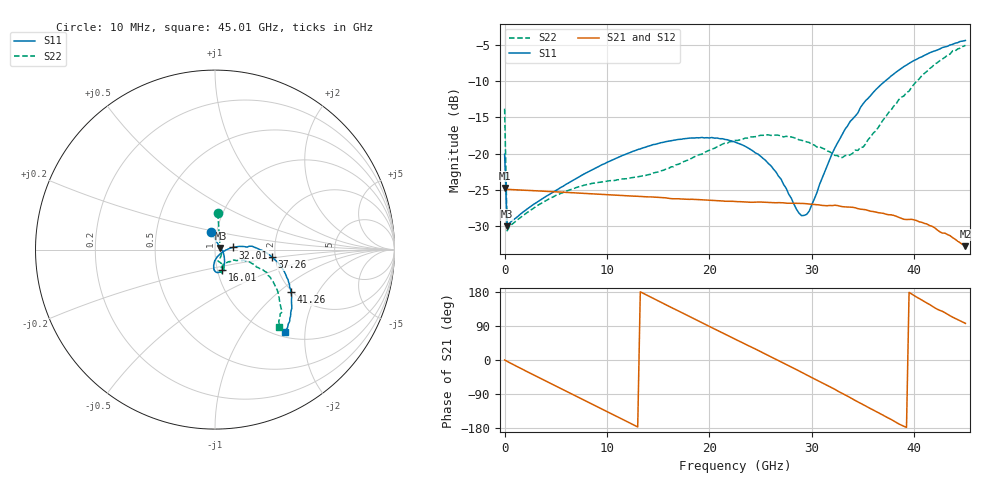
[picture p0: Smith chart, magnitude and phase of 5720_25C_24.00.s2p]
! Device:  ADRF5720
! Description: 0.5dB LSB GaAs MMIC 6-bit Digital Attenuator
! Frequency:  0.000009 -  40 GHz
! Ports:
!	RF1	= Port 1
!	RF2	= Port 2
! Vdd:  3.3 Volt
! Vss:  -3.3 Volt
! Control:  0/3.3 Volt
! State:  24.00 dB attenuation
! Data:  The device was measured using G-S-G Probes on a matrix board.
!  Data was collected using an calibrated 4 port network analyzer.
!  The reference plane for this measurement is at the launchers.
! Note:  Analog Devices supplies this data as a sample of measured data
!  for this product.  Your particular data for this product may vary.
!  Data was taken at 25 degrees C.
!  Analog Devices reserves the right to change this data at anytime.
# GHZ S DB R 45.0
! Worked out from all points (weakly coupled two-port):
!   181 points, 10 MHz to 45.01 GHz, reference 45 ohm
!   highest |S21| = -24.71 dB at 10 MHz (marker M1); lowest = -32.7 dB at 45.01 GHz (marker M2)
!   lowest |S11| = -30.0 dB at 260 MHz (marker M3), VSWR 1.07, Z = 47.8 + j0.88 ohm
!   |S11| at or under -10 dB: start of sweep to 37.17 GHz
!   |S22| runs from -30.6 to -5.1 dB; largest |S21 - S12| = 0.00012
!   S11 on the Smith chart (normalised r, x): 10 MHz: 0.94, +0.18; 16.01 GHz: 1.05, -0.25; 32.01 GHz: 1.22, +0.03; 37.26 GHz: 1.92, -0.18; 41.26 GHz: 1.97, -1.22; 45.01 GHz: 1.09, -1.57
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0.01  -20.08 103.8  -24.71 0.1  -24.71 0.1  -13.80 85.6
0.26  -30.01 16.9  -24.91 -3.8  -24.92 -3.8  -30.62 15.5
3.26  -26.59 -16.1  -25.12 -45.0  -25.13 -45.0  -27.10 -35.2
7.76  -22.80 -43.2  -25.47 -105.8  -25.47 -105.8  -24.35 -68.4
15.26  -18.49 -69.2  -26.04 152.5  -26.04 152.5  -22.38 -68.9
16.01  -18.28 -71.4  -26.14 142.2  -26.14 142.2  -22.06 -67.5
20.26  -17.77 -83.6  -26.43 85.2  -26.44 85.2  -19.36 -63.5
22.76  -18.54 -90.9  -26.61 51.9  -26.61 51.9  -18.18 -66.3
26.01  -21.65 -94.1  -26.73 8.4  -26.73 8.5  -17.48 -72.5
27.01  -23.50 -91.4  -26.75 -5.1  -26.75 -5.1  -17.58 -74.2
29.01  -28.54 -54.6  -26.85 -32.4  -26.85 -32.4  -18.16 -76.5
29.76  -27.90 -24.7  -26.94 -43.0  -26.94 -43.0  -18.46 -75.6
30.26  -26.23 -11.2  -27.00 -49.8  -27.00 -49.8  -18.81 -74.3
32.01  -19.94 6.9  -27.15 -73.7  -27.15 -73.6  -19.96 -66.6
33.01  -17.27 7.5  -27.30 -88.6  -27.30 -88.6  -20.52 -54.8
35.01  -13.14 3.4  -27.68 -117.3  -27.67 -117.3  -19.11 -33.3
37.26  -9.89 -7.5  -28.34 -150.0  -28.33 -150.0  -14.85 -20.1
37.76  -9.29 -10.2  -28.42 -156.9  -28.41 -156.9  -13.98 -19.7
39.76  -7.35 -21.2  -29.04 174.3  -29.04 174.4  -10.84 -22.7
41.26  -6.29 -29.1  -29.69 150.1  -29.72 150.1  -8.65 -28.9
43.76  -4.94 -42.5  -31.56 113.1  -31.55 113.1  -5.84 -42.9
45.01  -4.40 -49.7  -32.74 96.7  -32.74 96.7  -5.08 -50.3
